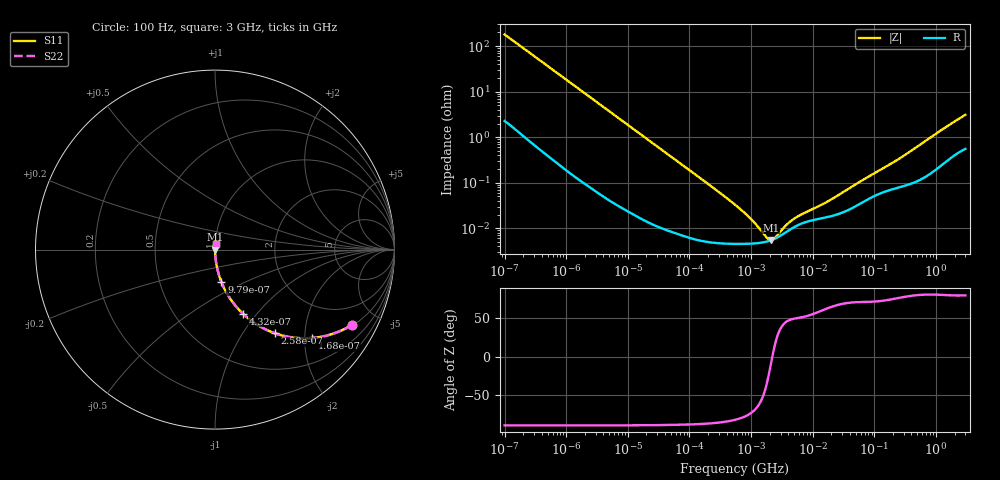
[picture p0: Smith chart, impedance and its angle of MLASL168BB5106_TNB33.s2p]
! MLASL168BB5106_TNB33  S-PARAMETER MODEL  ( Standard Model )
! Model Generated by TAIYO YUDEN Corporation (http://www.ty-top.com)
! Version 2.0
! TAIYO YUDEN Control No. 230906
! Copyright(c) 2012 TAIYO YUDEN CO.,LTD. All Rights Reserved.
! Product Description (link to TY-COMPAS)
! https://ds.yuden.co.jp/TYCOMPAS/or/detail?pn=MLASL168BB5106KTNB33&u=M
! Products Name : Multilayer Ceramic Capacitors
! Characteristics :
!  Capacitance : 10 [uF] , Rated Voltage : 10 [V] , TCC : X5R
!  Case Size : 1.6 x 0.8 / 0.063 x 0.031 [mm/inch] , Thickness : 0.8 / 0.031 [mm/inch]
!  (Conditions: Temperature = 25 [degC] , DC Bias Voltage = 0 [V])
! External Node Assignments :
!  1  o---| |---o  2
! GND o---------o GND
! Frequency Range : 100Hz  -  3GHz  [ 401 STEP ]
# MHZ S RI R 50
! Freq[MHz].  S11 Real  S11 Imag  S21 Real  S21 Imag  S12 Real  S12 Imag  S22 Real  S22 Imag
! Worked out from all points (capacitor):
!   401 points, 100 Hz to 3 GHz, reference 50 ohm
!   read as one part in series: C = 8.77 uF near 109 Hz
!   lowest |Z| = 5.52 mohm at 2.08 MHz (marker M1)
!   series resonance near 2.21 MHz, so ESL is about 590 pH
!   S11 on the Smith chart (normalised r, x): 100 Hz: 1.05, -3.62; 168 Hz: 1.03, -2.17; 258 Hz: 1.02, -1.42; 432 Hz: 1.01, -0.85; 979 Hz: 1.00, -0.38; 3 GHz: 1.01, +0.06
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0.0001  0.7632 -0.4189  0.2368 0.4189  0.2368 0.4189  0.7632 -0.4189
0.000119  0.6973 -0.4532  0.3027 0.4532  0.3027 0.4532  0.6973 -0.4532
0.000168  0.5402 -0.4924  0.4598 0.4924  0.4598 0.4924  0.5402 -0.4924
0.000258  0.3355 -0.4665  0.6645 0.4665  0.6645 0.4665  0.3355 -0.4665
0.000432  0.1549 -0.3564  0.8451 0.3564  0.8451 0.3564  0.1549 -0.3564
0.000636  0.0791 -0.2647  0.9209 0.2647  0.9209 0.2647  0.0791 -0.2647
0.000979  0.0358 -0.1809  0.9642 0.1809  0.9642 0.1809  0.0358 -0.1809
0.001788  0.0116 -0.102  0.9884 0.102  0.9884 0.102  0.0116 -0.102
0.005476  0.00153 -0.0339  0.9985 0.0339  0.9985 0.0339  0.00153 -0.0339
0.031977  0.00014 -0.00588  0.9999 0.00588  0.9999 0.00588  0.00014 -0.00588
0.547723  4.56e-05 -0.000327  1 0.000327  1 0.000327  4.56e-05 -0.000327
0.842342  4.57e-05 -0.000194  1 0.000194  1 0.000194  4.57e-05 -0.000194
1.352413  4.77e-05 -8.86e-05  1 8.86e-05  1 8.86e-05  4.77e-05 -8.86e-05
1.473992  4.84e-05 -7.21e-05  1 7.21e-05  1 7.21e-05  4.84e-05 -7.21e-05
2.079876  5.42e-05 -1.04e-05  0.9999 1.04e-05  0.9999 1.04e-05  5.42e-05 -1.04e-05
3.198641  7.26e-05 6.1e-05  0.9999 -6.1e-05  0.9999 -6.1e-05  7.26e-05 6.1e-05
5.361412  0.000112 0.000133  0.9999 -0.000133  0.9999 -0.000133  0.000112 0.000133
9.794414  0.00015 0.000214  0.9999 -0.000214  0.9999 -0.000214  0.00015 0.000214
19.50129  0.000183 0.000381  0.9998 -0.000381  0.9998 -0.000381  0.000183 0.000381
175.1444  0.000692 0.00239  0.9993 -0.00239  0.9993 -0.00239  0.000692 0.00239
1506.733  0.00329 0.017  0.9967 -0.017  0.9967 -0.017  0.00329 0.017
3000  0.00645 0.0303  0.9935 -0.0303  0.9935 -0.0303  0.00645 0.0303
